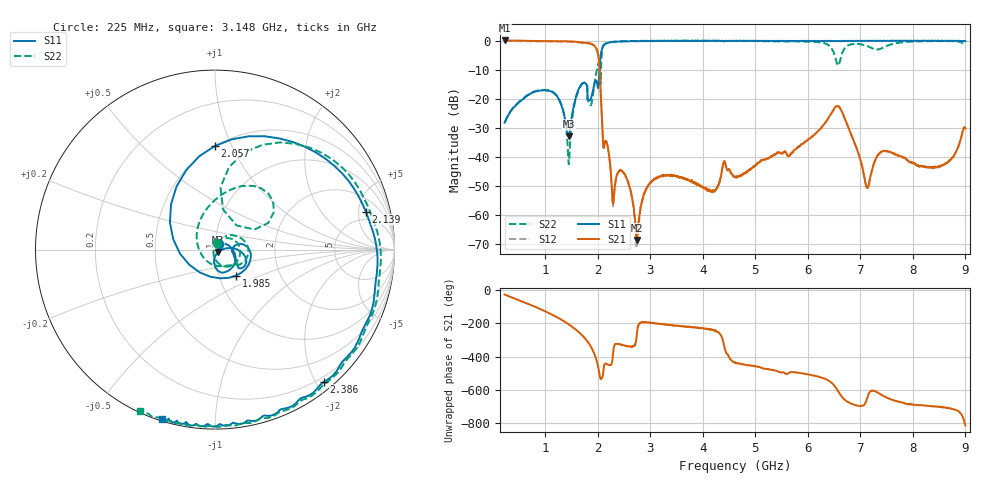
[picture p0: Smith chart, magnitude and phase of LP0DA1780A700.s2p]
!Agilent Technologies,E8358A,US41080443,A.07.50.56
!Agilent E8358A: A.07.50.56
!Date: Wednesday, August 24, 2016 14:53:27
!Correction: S11(Full 2 Port(1,2))
!S21(Full 2 Port(1,2))
!S12(Full 2 Port(1,2))
!S22(Full 2 Port(1,2))
!S2P File: Measurements: S11, S21, S12, S22:
# Hz S  dB  R 50
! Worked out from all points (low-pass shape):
!   1601 points, 225 MHz to 9 GHz, reference 50 ohm
!   highest |S21| = 0.03 dB at 225 MHz (marker M1); lowest = -68.5 dB at 2.748 GHz (marker M2)
!   |S21| within 3 dB of the highest: start of sweep to 1.977 GHz
!   lowest |S11| = -32.9 dB at 1.443 GHz (marker M3), VSWR 1.05, Z = 51.6 - j1.61 ohm
!   |S11| at or under -10 dB: start of sweep to 2.032 GHz
!   |S22| runs from -42.5 to 0.0 dB; largest |S21 - S12| = 0.019
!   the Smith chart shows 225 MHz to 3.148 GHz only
!   S11 on the Smith chart (normalised r, x): 225 MHz: 1.05, +0.06; 1.985 GHz: 1.21, -0.36; 2.057 GHz: 0.50, +0.87; 2.139 GHz: 3.54, +6.01; 2.386 GHz: 0.13, -2.11; 3.148 GHz: 0.01, -0.73
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2.25e8  -28.24 51.5  0.03 -27.3  -0.12 -27.1  -28.13 73.5
8.557031e8  -17.30 -39.3  -0.16 -107.4  -0.31 -107.2  -17.19 4.2
1.442531e9  -32.89 -43.6  -0.27 155.0  -0.42 155.2  -41.84 -166.6
1.689328e9  -15.02 -15.2  -0.65 92.4  -0.79 92.6  -15.20 13.9
1.881281e9  -19.19 10.2  -1.17 12.9  -1.31 13.1  -21.61 -169.7
1.985484e9  -14.56 -50.9  -3.34 -72.4  -3.48 -72.0  -9.74 79.3
2.056781e9  -4.77 90.0  -18.78 -174.5  -18.93 -174.3  -12.86 78.7
2.139047e9  -1.25 14.2  -34.61 -81.5  -34.78 -81.1  -1.07 16.2
2.385844e9  -0.40 -50.5  -45.40 36.7  -45.46 37.0  -0.30 -49.7
2.747812e9  -0.14 -86.2  -68.52 103.2  -69.38 115.1  -0.10 -88.9
3.148172e9  -0.10 -107.4  -46.80 157.3  -47.06 158.0  -0.07 -114.8
3.153656e9  -0.13 -107.7  -46.88 158.0  -47.14 158.4  -0.09 -115.0
4.6125e9  -0.15 -144.2  -46.85 -75.6  -46.86 -74.9  -0.13 174.8
6.076828e9  -0.08 -178.0  -32.96 -151.0  -33.25 -150.4  -0.47 68.0
6.427828e9  -0.21 173.7  -25.59 169.7  -25.63 170.4  -2.04 7.3
6.636234e9  -0.23 170.0  -23.98 85.0  -24.10 85.2  -5.28 150.7
6.80625e9  -0.11 165.7  -31.46 41.4  -31.61 42.0  -1.45 72.8
7.107891e9  -0.06 160.8  -50.12 50.8  -49.99 50.1  -1.78 -3.2
7.310812e9  -0.04 158.1  -39.94 108.7  -40.30 108.7  -3.10 -95.8
7.541156e9  -0.17 154.7  -38.23 69.5  -38.31 69.4  -1.61 162.8
7.985391e9  -0.08 150.1  -41.78 34.7  -42.14 34.1  -0.40 99.8
9e9  -0.15 139.3  -30.19 -91.9  -30.35 -92.3  -1.49 58.4
